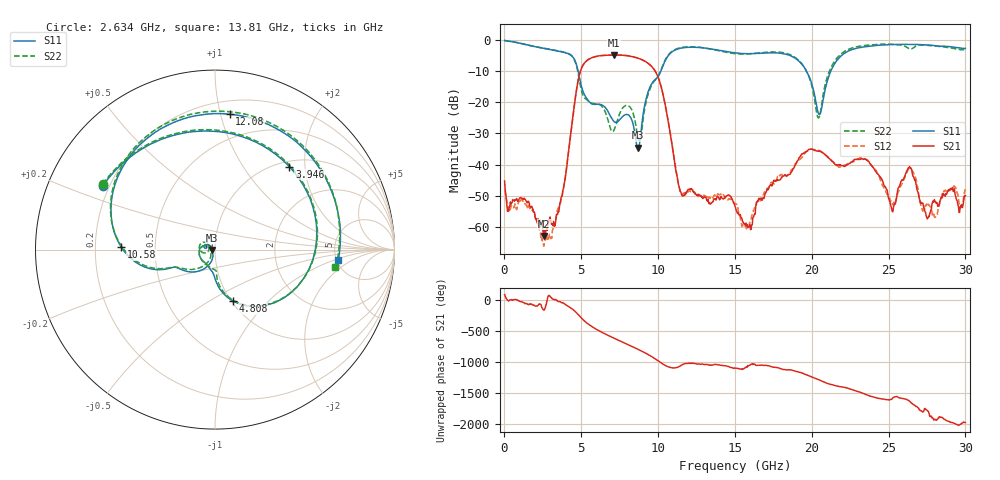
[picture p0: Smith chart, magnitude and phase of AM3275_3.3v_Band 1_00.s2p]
!Keysight Technologies,N5245B,MY58422270,A.16.20.02
!Date: Thursday, March 27, 2025 01:42:44
!Correction: S11(C  2-Port  )
!S21(C  2-Port  )
!S12(C  2-Port  )
!S22(C  2-Port  )
!S2P File: Measurements: S11, S21, S12, S22:
# Hz S  dB  R 50
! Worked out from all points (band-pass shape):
!   801 points, 10 MHz to 30 GHz, reference 50 ohm
!   highest |S21| = -4.88 dB at 7.133 GHz (marker M1); lowest = -62.9 dB at 2.559 GHz (marker M2)
!   |S21| within 3 dB of the highest: 5.146 GHz to 9.432 GHz (4.287 GHz wide, 58.8 % of centre)
!   lowest |S11| = -34.6 dB at 8.67 GHz (marker M3), VSWR 1.04, Z = 48.2 - j0.137 ohm
!   |S11| at or under -10 dB: 4.791 GHz to 10.18 GHz (5.392 GHz wide, 72 % of centre); 19.65 GHz to 21.24 GHz (1.595 GHz wide, 7.8 % of centre)
!   |S22| runs from -32.4 to -0.3 dB; largest |S21 - S12| = 0.0086
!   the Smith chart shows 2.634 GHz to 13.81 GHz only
!   S11 on the Smith chart (normalised r, x): 2.634 GHz: 0.17, +0.26; 3.946 GHz: 1.10, +1.66; 4.808 GHz: 1.02, -0.64; 10.58 GHz: 0.31, +0.01; 12.08 GHz: 0.30, +1.07; 13.81 GHz: 5.17, -1.15
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1e7  -0.23 -5.2  -45.23 88.1  -48.24 -46.4  -0.26 -5.9
1.022162e9  -1.10 -92.0  -50.51 -23.9  -52.20 -33.1  -1.12 -92.2
2.55915e9  -2.79 155.5  -62.85 -159.6  -66.13 136.9  -2.74 154.9
2.634125e9  -2.86 150.4  -61.81 -138.4  -64.74 10.1  -2.81 149.7
3.946188e9  -4.14 48.1  -44.79 -69.0  -44.27 -67.8  -4.07 47.1
4.8084e9  -10.39 -71.0  -12.73 123.6  -12.74 123.3  -11.12 -73.7
5.033325e9  -15.32 -88.9  -8.90 63.5  -8.90 63.4  -16.68 -86.3
5.895538e9  -20.72 -133.3  -5.43 -98.0  -5.43 -98.1  -20.47 -134.4
7.132625e9  -26.23 161.9  -4.88 106.5  -4.88 106.4  -28.97 -171.8
8.669612e9  -34.60 -175.6  -5.87 -69.0  -5.87 -69.0  -31.12 153.4
1.001916e10  -11.63 -157.4  -12.24 100.1  -12.23 100.0  -11.43 -157.9
1.058148e10  -5.64 178.4  -24.00 15.0  -23.97 15.5  -5.45 176.0
1.208098e10  -2.40 83.8  -47.76 61.9  -48.30 61.1  -2.24 81.9
1.38054e10  -3.23 -4.9  -50.87 43.6  -49.90 44.2  -3.37 -8.4
1.5005e10  -4.21 -74.5  -53.33 -13.5  -52.45 -9.5  -4.46 -79.4
1.687938e10  -4.27 176.7  -50.90 26.7  -49.39 33.0  -4.07 173.2
2.002832e10  -14.57 15.9  -35.02 -159.1  -35.11 -158.3  -15.22 15.8
2.182772e10  -5.55 136.3  -40.27 47.9  -40.77 47.3  -4.90 133.4
2.501416e10  -1.60 38.9  -50.98 -166.4  -50.48 -158.7  -1.41 36.5
2.636371e10  -1.50 6.8  -40.63 172.9  -41.57 170.7  -2.93 4.7
2.748834e10  -1.66 -22.8  -56.95 33.2  -52.87 -81.7  -1.79 -22.2
3e10  -2.78 -111.2  -49.98 -169.7  -47.86 -159.4  -3.15 -111.5
